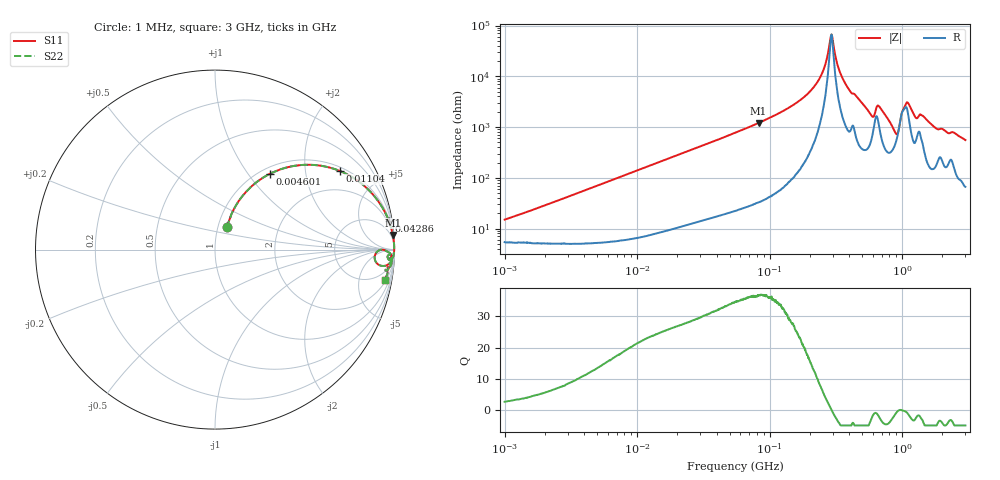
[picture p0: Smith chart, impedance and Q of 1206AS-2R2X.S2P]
!s-Parameter Generated by FASTRON Sdn. Bhd.
!FASTRON P/N : 1206AS-2R2X
!Keysight Technologies: E4991B_MY54100416_A.01.15
!Date created: Thu Nov 16 13:47:41 2023
!Version  : Rev00 Thu Nov 16 13:47:41 2023
!Data & Calibration Information:
!Freq	S11	S21	S12	S22
!PortZ  Port1:50+j0  Port2:50+j0
!When reading reference impedance value at option line is always used.
! Remarks : This data is being provided solely for informational purposes.
# Hz S dB R 50
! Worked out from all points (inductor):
!   1601 points, 1 MHz to 3 GHz, reference 50 ohm
!   read as one part in series: L = 2.23 uH near 1.145 MHz
!   highest Q = 36.8 at 82.56 MHz (marker M1), where L = 2.32 uH
!   self-resonance near 291.3 MHz
!   S11 on the Smith chart (normalised r, x): 1 MHz: 1.11, +0.28; 4.601 MHz: 1.10, +1.28; 11.04 MHz: 1.14, +3.07; 42.86 MHz: 1, +12; 3 GHz: 2, -11
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1000000  -17.01 61.3  -0.53 -7.6  -0.53 -7.6  -17.01 61.3
3804036  -6.87 57.8  -1.41 -26.8  -1.41 -26.8  -6.87 57.8
4600725  -5.63 54.0  -1.81 -31.4  -1.81 -31.4  -5.63 54.0
1.104425e7  -1.71 32.3  -5.44 -55.1  -5.44 -55.1  -1.71 32.3
1.447069e7  -1.10 26.0  -7.16 -61.7  -7.16 -61.7  -1.10 26.0
4.286213e7  -0.16 9.5  -15.65 -78.7  -15.65 -78.7  -0.16 9.5
5.477226e7  -0.11 7.4  -17.80 -80.9  -17.80 -80.9  -0.11 7.4
8.255875e7  -0.05 4.7  -21.66 -83.7  -21.66 -83.7  -0.05 4.7
2.083556e8  -0.01 1.0  -34.85 -84.9  -34.85 -84.9  -0.01 1.0
2.519921e8  -0.01 0.5  -41.91 -79.6  -41.91 -79.6  -0.01 0.5
2.92808e8  -0.01 -0.0  -56.49 0.6  -56.49 0.6  -0.01 -0.0
3.368469e8  -0.02 -0.4  -42.04 76.9  -42.04 76.9  -0.02 -0.4
4.013235e8  -0.03 -1.1  -34.36 79.9  -34.36 79.9  -0.03 -1.1
5.870266e8  -0.19 -3.1  -24.69 66.9  -24.69 66.9  -0.19 -3.1
6.652545e8  -0.15 -1.9  -28.47 62.0  -28.47 62.0  -0.15 -1.9
7.925923e8  -0.17 -4.0  -22.82 72.8  -22.82 72.8  -0.17 -4.0
9.117997e8  -0.95 -4.1  -18.12 31.3  -18.12 31.3  -0.95 -4.1
1.023018e9  -0.36 -0.7  -27.39 16.0  -27.39 16.0  -0.36 -0.7
1.097256e9  -0.19 -1.3  -29.91 46.0  -29.91 46.0  -0.19 -1.3
1.268618e9  -0.22 -3.4  -23.84 65.8  -23.84 65.8  -0.22 -3.4
1.402151e9  -0.18 -3.1  -24.81 68.1  -24.81 68.1  -0.18 -3.1
3e9  -0.32 -10.0  -15.18 73.2  -15.18 73.2  -0.32 -10.0
